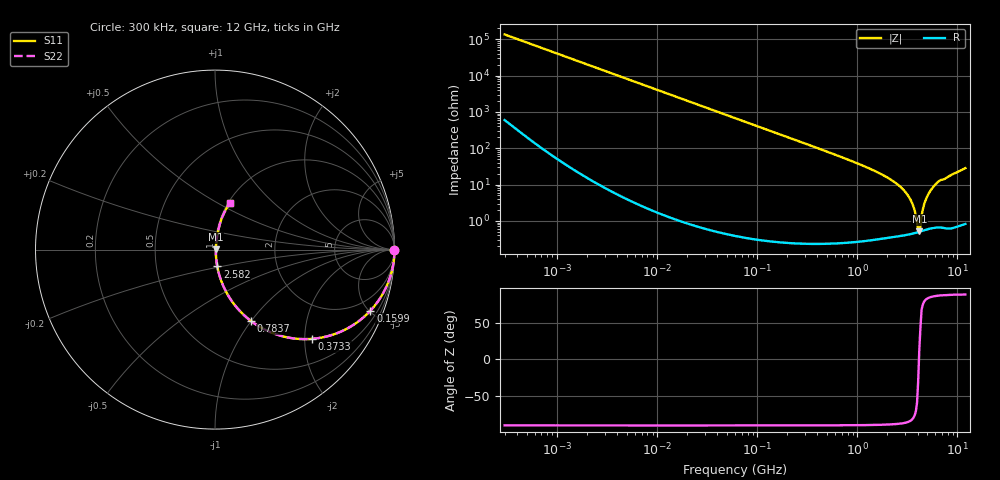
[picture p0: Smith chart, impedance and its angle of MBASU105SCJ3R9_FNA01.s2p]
! MBASU105SCJ3R9_FNA01  S-PARAMETER MODEL  ( Standard Model )
! Model Generated by TAIYO YUDEN Corporation (http://www.ty-top.com)
! Version 1.0
! TAIYO YUDEN Control No. 230609
! Copyright(c) 2023 TAIYO YUDEN CO.,LTD. All Rights Reserved.
! Product Description (link to TY-COMPAS)
! https://ds.yuden.co.jp/TYCOMPAS/or/detail?pn=MBASU105SCJ3R9CFNA01&u=M
! Products Name : Multilayer Ceramic Capacitors
! Characteristics :
!  Capacitance : 3.9 [pF] , Rated Voltage : 50 [V] , TCC : CJ / C0J
!  Case Size : 1.0 x 0.5 / 0.039 x 0.02 [mm/inch] , Thickness : 0.5 / 0.02 [mm/inch]
!  (Conditions: Temperature = 25 [degC] , DC Bias Voltage = 0 [V])
! External Node Assignments :
!  1  o---| |---o  2
! GND o---------o GND
! Frequency Range : 0.3MHz  -  12000MHz  [ 401 STEP ]
# MHZ S RI R 50
! Freq[MHz].  S11 Real  S11 Imag  S21 Real  S21 Imag  S12 Real  S12 Imag  S22 Real  S22 Imag
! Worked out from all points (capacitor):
!   401 points, 300 kHz to 12 GHz, reference 50 ohm
!   read as one part in series: C = 3.9 pF near 316.3 kHz
!   lowest |Z| = 515 mohm at 4.159 GHz (marker M1)
!   series resonance near 4.127 GHz, so ESL is about 380 pH
!   S11 on the Smith chart (normalised r, x): 300 kHz: open; 159.9 MHz: 1.01, -5.10; 373.3 MHz: 1.00, -2.17; 783.7 MHz: 1.00, -1.00; 2.582 GHz: 1.01, -0.19; 12 GHz: 1.02, +0.57
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0.3  1 -0.000735  3.77e-06 0.000735  3.77e-06 0.000735  1 -0.000735
1.769972  1 -0.00434  2.23e-05 0.00434  2.23e-05 0.00434  1 -0.00434
10.44266  0.9993 -0.0256  0.000665 0.0256  0.000665 0.0256  0.9993 -0.0256
60  0.9788 -0.1439  0.0212 0.1439  0.0212 0.1439  0.9788 -0.1439
159.8975  0.8663 -0.3398  0.1337 0.3398  0.1337 0.3398  0.8663 -0.3398
353.9943  0.5668 -0.4945  0.4332 0.4945  0.4332 0.4945  0.5668 -0.4945
373.2558  0.5403 -0.4973  0.4597 0.4973  0.4597 0.4973  0.5403 -0.4973
783.7017  0.2023 -0.3993  0.7977 0.3993  0.7977 0.3993  0.2023 -0.3993
1366.97  0.0682 -0.2467  0.9318 0.2467  0.9318 0.2467  0.0682 -0.2467
2088.533  0.0238 -0.141  0.9762 0.141  0.9762 0.141  0.0238 -0.141
2581.562  0.0127 -0.0941  0.9873 0.0941  0.9873 0.0941  0.0127 -0.0941
3364.605  0.00584 -0.0395  0.9942 0.0395  0.9942 0.0395  0.00584 -0.0395
3642.919  0.00506 -0.0237  0.9949 0.0237  0.9949 0.0237  0.00506 -0.0237
3944.255  0.00484 -0.00803  0.9952 0.00803  0.9952 0.00803  0.00484 -0.00803
4050.141  0.00489 -0.00281  0.9951 0.00281  0.9951 0.00281  0.00489 -0.00281
4158.869  0.00499 0.00117  0.995 -0.00117  0.995 -0.00117  0.00499 0.00117
4270.516  0.00512 0.00494  0.9949 -0.00494  0.9949 -0.00494  0.00512 0.00494
4623.766  0.00615 0.0262  0.9939 -0.0262  0.9939 -0.0262  0.00615 0.0262
4875.354  0.00733 0.0402  0.9927 -0.0402  0.9927 -0.0402  0.00733 0.0402
5715.274  0.0134 0.0836  0.9866 -0.0836  0.9866 -0.0836  0.0134 0.0836
6699.894  0.023 0.1267  0.977 -0.1267  0.977 -0.1267  0.023 0.1267
12000  0.0808 0.2585  0.9192 -0.2585  0.9192 -0.2585  0.0808 0.2585
